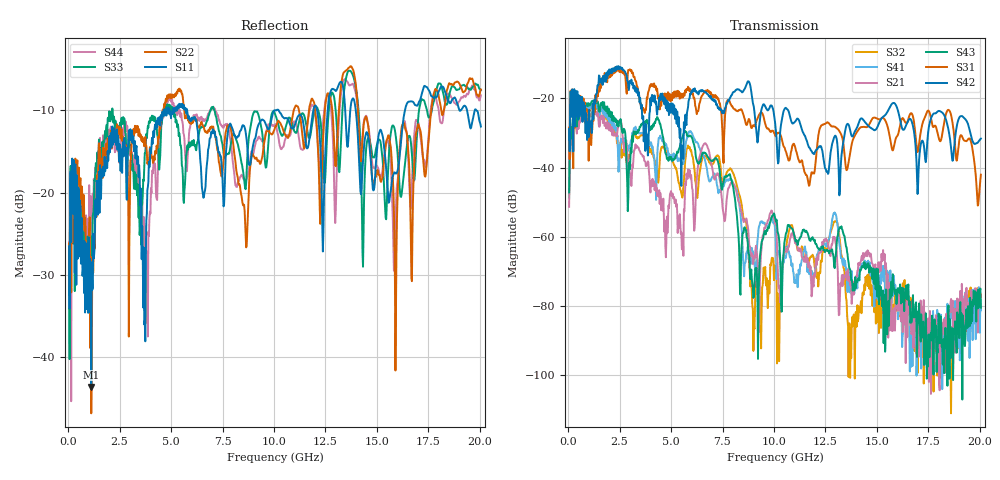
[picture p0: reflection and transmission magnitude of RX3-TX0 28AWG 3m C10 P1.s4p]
! FILE: O:\PROJECTS\SI-2007-05-003 3m Eyemax Qual\XT\FD\RX0-TX1 28AWG 3m C10 P1.s4p
# MHZ S RI R 50.00
! FREQ  S11  S12  S13  S14
!  S21  S22  S23  S24
!  S31  S32  S33  S34
!  S41  S42  S43  S44
!  REAL  IMAG  REAL  IMAG  REAL  IMAG  REAL  IMAG
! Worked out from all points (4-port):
!   801 points, 50 MHz to 20.05 GHz, reference 50 ohm
!   strongest paths, dB at 50 MHz, 5.05 GHz, 10.05 GHz, 15.05 GHz, 20.05 GHz:
!     S42: -28.8, -24.2, -26.8, -27.9, -31.7
!     S31: -28.5, -20.5, -30.6, -26.0, -42.1
!     S43: -47.2, -38.1, -54.5, -69.3, -80.5
!     S21: -51.3, -48.3, -56.0, -72.1, -80.2
!     S41: -48.8, -36.4, -57.5, -78.1, -81.2
!     S32: -47.7, -37.9, -68.3, -75.5, -77.5
!   lowest |S11| = -43.7 dB at 1.125 GHz (marker M1), VSWR 1.01, Z = 50.2 - j0.616 ohm
!   |S11| at or under -10 dB: start of sweep to 4.646 GHz; 5.783 GHz to 10.01 GHz (4.23 GHz wide, 53.6 % of centre); 13.97 GHz to 16.36 GHz (2.385 GHz wide, 15.7 % of centre)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
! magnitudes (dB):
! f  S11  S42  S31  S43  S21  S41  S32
! 50 MHz  -26.5  -28.8  -28.5  -47.2  -51.3  -48.8  -47.7
! 1.125 GHz  -43.7  -26.6  -33.5  -21.1  -24.5  -22.2  -22.6
! 4.75 GHz  -10.2  -22.9  -20.8  -36.1  -65.9  -33.1  -35.1
! 7.95 GHz  -12.0  -19.1  -22.3  -43.9  -44.3  -43.7  -40.7
! 9.025 GHz  -13.8  -22.6  -27.9  -77.3  -65.6  -65.8  -84.9
! 12.97 GHz  -7.6  -30.8  -28.3  -66.0  -61.0  -53.2  -55.6
! 20.05 GHz  -12.0  -31.7  -42.1  -80.5  -80.2  -81.2  -77.5
